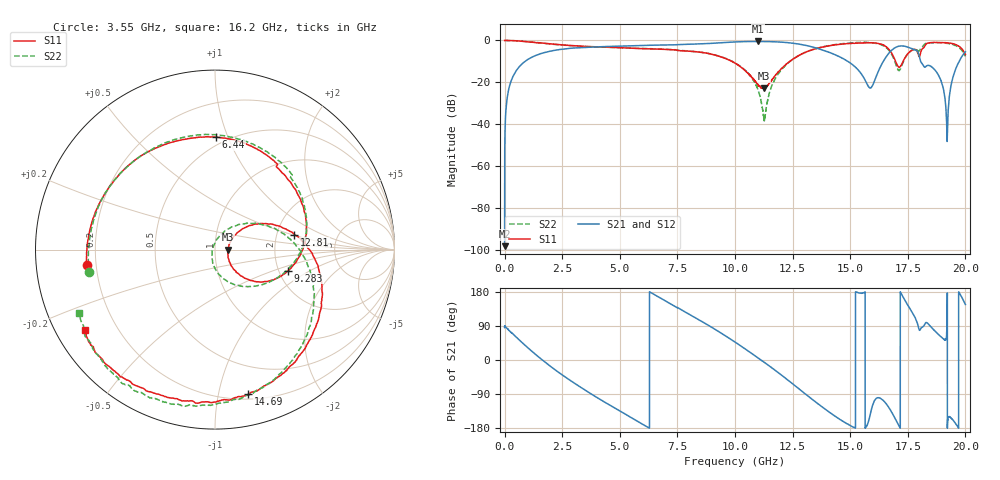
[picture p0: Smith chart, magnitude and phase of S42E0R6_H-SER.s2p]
!{S42E0R6}
!Johanson Technology Inc.
!www.johansontechnology.com
!Test Board Conditions:
!Substrate Type  RO4350B
!Substrate Thickness  50 mil
!Substrate Dk  3.66
!TL Type: GCPW
!TL Trace Width  60 mil
!TL Gap  10 mil
!Electrode orientation  Horizontal
!DUT TOPOLOGY	SERIES
!Mounting Pad LxW  14x55 mil
! Created Wed Nov 25 21:26:50 2020
# khz S ma R 50
! 2 Port Network Data from SP1.SP block
! freq  magS11  angS11  magS21  angS21  magS12  angS12  magS22  angS22
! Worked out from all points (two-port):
!   20001 points, 300 kHz to 20 GHz, reference 50 ohm
!   highest |S21| = -0.47 dB at 11.01 GHz (marker M1); lowest = -98.1 dB at 300 kHz (marker M2)
!   |S21| within 3 dB of the highest: 3.202 GHz to 13.49 GHz (10.29 GHz wide, 123 % of centre); 16.94 GHz to 17.58 GHz (633.4 MHz wide, 3.67 % of centre)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
!   lowest |S11| = -22.9 dB at 11.26 GHz (marker M3), VSWR 1.15, Z = 57.7 - j0.0286 ohm
!   |S11| at or under -10 dB: 9.871206 GHz to 9.874214 GHz (3.009 MHz wide, 0.0305 % of centre); 9.874 GHz to 12.37 GHz (2.498 GHz wide, 22.5 % of centre); 16.97 GHz to 17.3 GHz (325.6 MHz wide, 1.9 % of centre)
!   |S22| runs from -38.3 to 0.0 dB; largest |S21 - S12| = 0.013
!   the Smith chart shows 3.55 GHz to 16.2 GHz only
!   S11 on the Smith chart (normalised r, x): 3.55 GHz: 0.16, -0.06; 6.44 GHz: 0.44, +0.91; 9.283 GHz: 2.25, -0.64; 12.81 GHz: 2.51, +0.53; 14.69 GHz: 0.24, -1.23; 16.2 GHz: 0.09, -0.28
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300  0.9985 -0.3  1.244e-05 86.6  0.0001422 83.9  1 -0.3
131300  0.9982 -7.8  0.05051 81.9  0.05086 81.8  0.9984 -7.7
506300  0.9808 -29.8  0.1906 60.4  0.1913 60.5  0.9808 -29.8
1640300  0.8661 -89.7  0.4986 -0.0  0.4996 -0.1  0.8617 -90.6
3334300  0.7289 -164.6  0.6768 -73.2  0.6762 -73.3  0.7263 -161.8
3550300  0.719 -173.3  0.6848 -81.5  0.6852 -81.6  0.7153 -169.8
6440300  0.6267 89.5  0.7706 174.7  0.7682 174.6  0.6324 80.6
6667300  0.6209 81.9  0.7756 166.8  0.7737 166.6  0.6262 72.4
9283300  0.4242 -16.1  0.8735 75.3  0.8782 75.5  0.428 -13.5
1.00003e7  0.2876 -38.2  0.9207 47.3  0.9212 47.4  0.291 -44.6
1.10133e7  0.08621 -32.1  0.9468 4.9  0.9453 4.9  0.06286 -103.1
1.12623e7  0.0717 -0.2  0.941 -5.8  0.9436 -5.7  0.01317 179.3
1.28143e7  0.4499 10.7  0.8133 -78.1  0.8118 -77.9  0.4503 3.4
1.33343e7  0.594 -12.1  0.7037 -103.1  0.7096 -103.0  0.5971 -22.7
1.46923e7  0.8258 -77.0  0.3701 -161.9  0.3701 -162.3  0.8429 -80.5
1.61963e7  0.8525 -148.6  0.1709 -99.6  0.1704 -99.1  0.835 -155.4
1.66673e7  0.6232 -177.5  0.4885 -124.5  0.4876 -123.8  0.5942 170.1
1.72073e7  0.2544 -141.1  0.7405 176.1  0.7367 176.3  0.2261 -145.1
1.78183e7  0.609 -158.8  0.5973 112.0  0.5974 112.8  0.6118 -159.6
1.88473e7  0.8858 160.1  0.1427 66.3  0.1421 66.4  0.8855 154.3
1.92033e7  0.8785 138.4  0.004567 105.0  0.004654 105.4  0.8544 133.9
2e7  0.4646 76.8  0.5358 146.4  0.5381 146.7  0.4173 80.6
